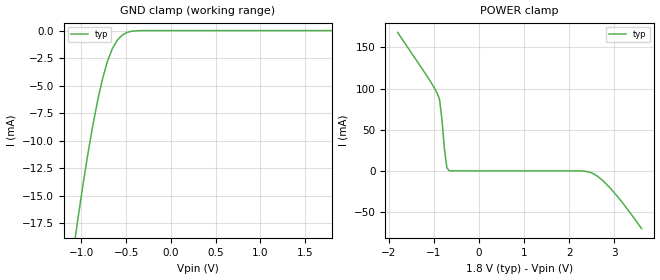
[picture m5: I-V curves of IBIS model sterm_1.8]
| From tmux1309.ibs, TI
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| sterm_1.8
[Model]   sterm_1.8
Model_type   Terminator
|   typ   min   max
C_comp   1.008417e-12   NA   NA
[Voltage Range]   1.8   NA   NA
[Temperature Range]   27   NA   NA
[Power Clamp Reference]   1.8   NA   NA
[GND Clamp Reference]   0   NA   NA
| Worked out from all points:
|   GND clamp passes 1 mA (typ) near -0.61 V on its own axis
|   POWER clamp passes 1 mA (typ) near -0.67 V on its own axis
[GND Clamp]
|   Voltage   I(typ)   I(min)   I(max)
-3.6V     -4.477kA   NA         NA
-1.091V   -20.1mA    NA         NA
-1.036V   -16.96mA   NA         NA
-927.3mV  -11.19mA   NA         NA
-872.7mV  -8.635mA   NA         NA
-818.2mV  -6.344mA   NA         NA
-763.6mV  -4.377mA   NA         NA
-709.1mV  -2.797mA   NA         NA
-654.5mV  -1.646mA   NA         NA
-545.5mV  -418.7uA   NA         NA
-327.3mV  -3.652uA   NA         NA
1.8V      463.6pA    NA         NA
[POWER Clamp]
|   Voltage   I(typ)   I(min)   I(max)
-1.8V     168.2mA    NA         NA
-1.091V   110.1mA    NA         NA
-927.3mV  94.67mA    NA         NA
-872.7mV  87.09mA    NA         NA
-818.2mV  62.28mA    NA         NA
-763.6mV  26.58mA    NA         NA
-709.1mV  3.618mA    NA         NA
-654.5mV  83.29uA    NA         NA
2.455V    -1.646mA   NA         NA
2.673V    -8.635mA   NA         NA
2.891V    -20.1mA    NA         NA
3.6V      -70.22mA   NA         NA
